(* Logix 5000 AddOnInstructionDefinition export AMCI_3202_AOP_Run_Blend; software revision 20.03 *)

ADD_ON_INSTRUCTION AMCI_3202_AOP_Run_Blend   (* revision 1.0, vendor AMCI, ExecuteEnableInFalse *)
VAR_INPUT
   axis_status_bits : INT; {required}
   channel_number : INT; {required}
   Direction_0_for_CW_1_for_CCW : BOOL; {required}
END_VAR
VAR_IN_OUT
   AMCI_3202_output_data : AM:1756_3202:O:0; {required}
END_VAR
VAR_OUTPUT
   EN : BOOL; {access Read Only, visible}
   ER : BOOL; {access Read Only, visible}
END_VAR
VAR
   command_data_block : DINT[8]; {access None}
END_VAR

ROUTINE EnableInFalse   (* ladder *)
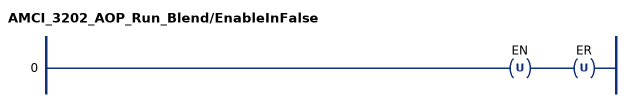
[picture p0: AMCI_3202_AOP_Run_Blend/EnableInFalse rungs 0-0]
   0: OTU(EN)OTU(ER);
END_ROUTINE

ROUTINE Logic   (* ladder *)
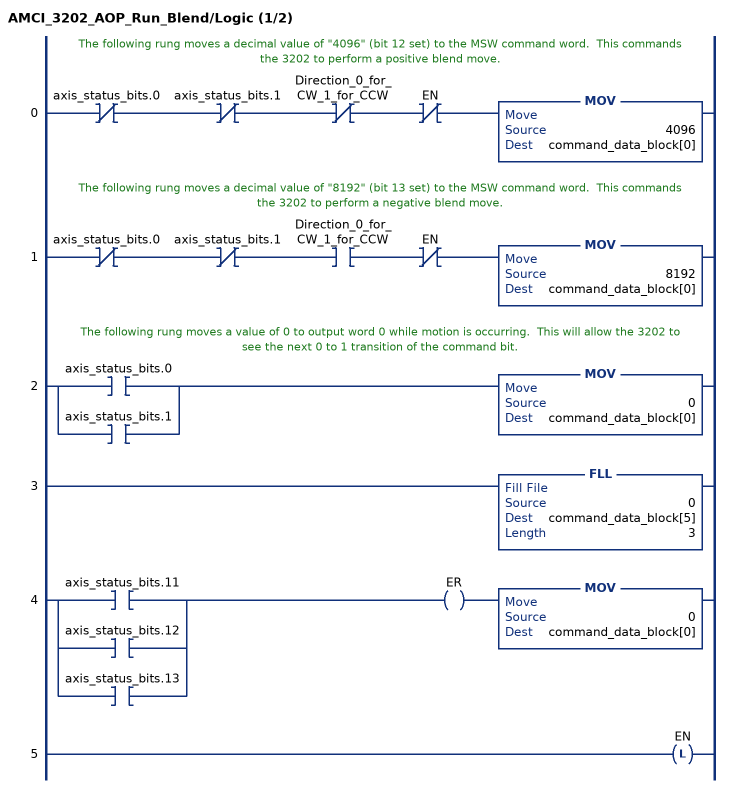
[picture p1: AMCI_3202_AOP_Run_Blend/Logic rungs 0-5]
   // The following rung moves a decimal value of "4096" (bit 12 set) to the MSW command word.  This commands the 3202 to perform a positive blend move.
   0: XIO(axis_status_bits.0)XIO(axis_status_bits.1)XIO(Direction_0_for_CW_1_for_CCW)XIO(EN)MOV(4096,command_data_block[0]);
   // The following rung moves a decimal value of "8192" (bit 13 set) to the MSW command word.  This commands the 3202 to perform a negative blend move.
   1: XIO(axis_status_bits.0)XIO(axis_status_bits.1)XIC(Direction_0_for_CW_1_for_CCW)XIO(EN)MOV(8192,command_data_block[0]);
   // The following rung moves a value of 0 to output word 0 while motion is occurring.  This will allow the 3202 to see the next 0 to 1 transition of the command bit.
   2: [XIC(axis_status_bits.0) ,XIC(axis_status_bits.1) ]MOV(0,command_data_block[0]);
   3: FLL(0,command_data_block[5],3);
   4: [XIC(axis_status_bits.11) ,XIC(axis_status_bits.12) ,XIC(axis_status_bits.13) ]OTE(ER)MOV(0,command_data_block[0]);
   5: OTL(EN);
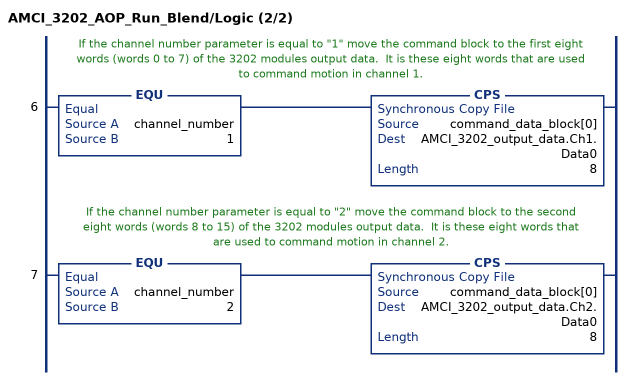
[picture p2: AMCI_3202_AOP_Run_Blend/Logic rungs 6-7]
   // If the channel number parameter is equal to "1" move the command block to the first eight words (words 0 to 7) of the 3202 modules output data.  It is these eight words that are used to command motion in channel 1.
   6: EQU(channel_number,1)CPS(command_data_block[0],AMCI_3202_output_data.Ch1.Data0,8);
   // If the channel number parameter is equal to "2" move the command block to the second eight words (words 8 to 15) of the 3202 modules output data.  It is these eight words that are used to command motion in channel 2.
   7: EQU(channel_number,2)CPS(command_data_block[0],AMCI_3202_output_data.Ch2.Data0,8);
END_ROUTINE
END_ADD_ON_INSTRUCTION
